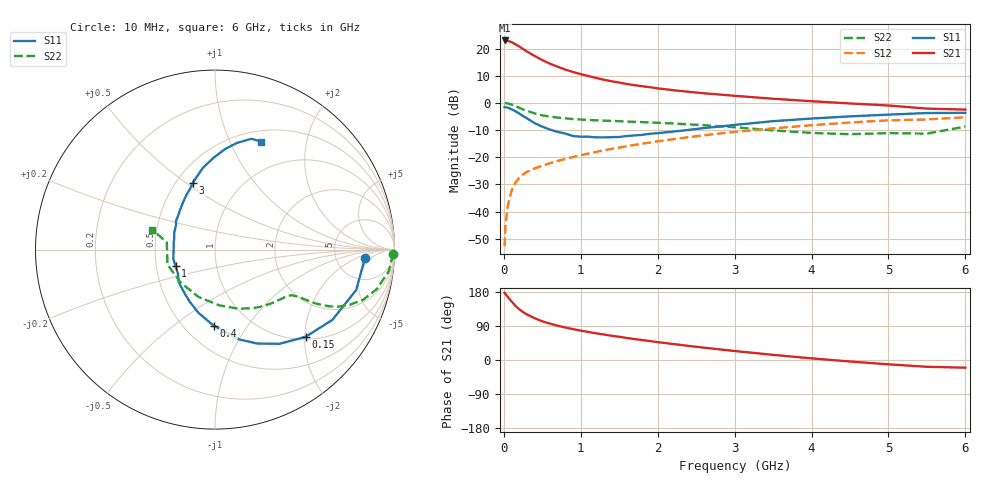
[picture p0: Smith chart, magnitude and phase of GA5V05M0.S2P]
! Infineon Technologies  Discrete & RF Semiconductors
! BF775
! Si NPN RF Bipolar Junction Transistor in SOT23
! VCE = 5 V  IC = 5 mA
! Common Emitter S-Parameters:  May  1996
# GHz  S  MA  R  50
!  f  S11  S21  S12  S22
! GHz  MAG  ANG  MAG  ANG  MAG  ANG  MAG  ANG
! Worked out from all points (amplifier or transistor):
!   36 points, 10 MHz to 6 GHz, reference 50 ohm
!   highest |S21| = 23.0 dB at 10 MHz (marker M1)
!   |S21| within 3 dB of that: start of sweep to 242.4 MHz
!   unconditionally stable (mu >= 1): 824.5 MHz to 3.196 GHz
!   at 250 MHz: K = 0.48, MSG = 23.1 dB, |S12| = -26.4 dB
!   at 1.4 GHz: K = 1.12, MAG = 10.4 dB, |S12| = -17.0 dB
!   at 6 GHz: K = 0.93, MSG = 1.4 dB, |S12| = -5.3 dB
!   lowest NFmin = 1.50 dB at 450 MHz
!   S11 on the Smith chart (normalised r, x): 10 MHz: 10, -3; 150 MHz: 1.06, -2.02; 400 MHz: 0.69, -0.71; 1 GHz: 0.63, -0.12; 3 GHz: 0.60, +0.53; 6 GHz: 0.63, +1.32
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0.01  0.8367 -3.1  14.09 177.4  0.0023 89.2  0.9939 -1.4
0.02  0.8285 -6.3  13.83 174.3  0.0051 84.6  0.9871 -2.9
0.05  0.8182 -16.0  13.88 166.7  0.0125 80.8  0.9754 -7.2
0.1  0.7622 -30.9  13.13 154.6  0.0242 73.9  0.9277 -13.7
0.15  0.7008 -43.9  11.98 143.1  0.0341 68.7  0.8717 -18.7
0.2  0.6362 -55.6  10.96 134.0  0.0414 64.5  0.8108 -22.3
0.25  0.5725 -66.0  9.807 126.4  0.0481 61.0  0.7551 -24.9
0.3  0.5193 -74.7  8.801 120.1  0.0537 59.2  0.7122 -26.4
0.4  0.4236 -91.0  7.309 110.3  0.062 57.2  0.6394 -28.1
0.5  0.3646 -104.6  6.114 102.0  0.0696 56.9  0.5887 -28.8
0.6  0.3221 -116.1  5.263 96.0  0.0775 56.6  0.5579 -29.2
0.8  0.2717 -138.1  4.095 85.7  0.0929 57.3  0.5182 -30.0
1  0.2379 -157.3  3.376 77.5  0.1087 58.4  0.4939 -31.1
1.1  0.238 -167.4  3.112 73.9  0.1168 58.5  0.4839 -32.2
1.3  0.2309 177.7  2.666 67.3  0.1337 58.5  0.4701 -34.3
1.6  0.2453 157.8  2.227 58.1  0.1591 57.7  0.4531 -38.3
2.2  0.2956 131.0  1.711 42.2  0.2143 54.7  0.4175 -48.6
3  0.3926 108.3  1.348 23.7  0.2916 47.6  0.3559 -68.0
3.5  0.4602 98.5  1.191 13.6  0.3393 42.0  0.3114 -85.5
4.5  0.5641 84.1  0.975 -4.0  0.4352 29.5  0.2652 -135.7
5.5  0.6499 71.8  0.784 -17.9  0.4952 14.4  0.2714 171.5
6  0.6549 66.7  0.752 -20.3  0.5437 10.1  0.3664 162.3
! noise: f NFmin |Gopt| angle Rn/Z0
0.45  1.5  0.28  29  0.34
0.9  1.8  0.25  59  0.34
